DATA_BLOCK DB 6
TITLE =Codici trasferitore SALVARE PRIMA DEL DOWNLOAD
VERSION : 0.1


  STRUCT
   Codici : ARRAY  [0 .. 200 ] OF WORD ;
  END_STRUCT ;
BEGIN
   Codici[0] := W#16#FFFF;
   Codici[1] := W#16#FFFF;
   Codici[2] := W#16#DB;
   Codici[3] := W#16#FFFF;
   Codici[4] := W#16#4;
   Codici[5] := W#16#FFFF;
   Codici[6] := W#16#3;
   Codici[7] := W#16#DC;
   Codici[8] := W#16#9;
   Codici[9] := W#16#8;
   Codici[10] := W#16#D9;
   Codici[11] := W#16#0;
   Codici[12] := W#16#DA;
   Codici[13] := W#16#0;
   Codici[14] := W#16#0;
   Codici[15] := W#16#0;
   Codici[16] := W#16#0;
   Codici[17] := W#16#0;
   Codici[18] := W#16#0;
   Codici[19] := W#16#0;
   Codici[20] := W#16#0;
   Codici[21] := W#16#0;
   Codici[22] := W#16#0;
   Codici[23] := W#16#0;
   Codici[24] := W#16#0;
   Codici[25] := W#16#0;
   Codici[26] := W#16#0;
   Codici[27] := W#16#0;
   Codici[28] := W#16#0;
   Codici[29] := W#16#0;
   Codici[30] := W#16#0;
   Codici[31] := W#16#0;
   Codici[32] := W#16#0;
   Codici[33] := W#16#0;
   Codici[34] := W#16#0;
   Codici[35] := W#16#0;
   Codici[36] := W#16#0;
   Codici[37] := W#16#0;
   Codici[38] := W#16#0;
   Codici[39] := W#16#0;
   Codici[40] := W#16#0;
   Codici[41] := W#16#0;
   Codici[42] := W#16#0;
   Codici[43] := W#16#0;
   Codici[44] := W#16#0;
   Codici[45] := W#16#0;
   Codici[46] := W#16#0;
   Codici[47] := W#16#0;
   Codici[48] := W#16#0;
   Codici[49] := W#16#0;
   Codici[50] := W#16#0;
   Codici[51] := W#16#0;
   Codici[52] := W#16#0;
   Codici[53] := W#16#0;
   Codici[54] := W#16#0;
   Codici[55] := W#16#0;
   Codici[56] := W#16#0;
   Codici[57] := W#16#0;
   Codici[58] := W#16#0;
   Codici[59] := W#16#0;
   Codici[60] := W#16#0;
   Codici[61] := W#16#0;
   Codici[62] := W#16#0;
   Codici[63] := W#16#0;
   Codici[64] := W#16#0;
   Codici[65] := W#16#0;
   Codici[66] := W#16#0;
   Codici[67] := W#16#0;
   Codici[68] := W#16#0;
   Codici[69] := W#16#0;
   Codici[70] := W#16#0;
   Codici[71] := W#16#0;
   Codici[72] := W#16#0;
   Codici[73] := W#16#0;
   Codici[74] := W#16#0;
   Codici[75] := W#16#0;
   Codici[76] := W#16#0;
   Codici[77] := W#16#0;
   Codici[78] := W#16#0;
   Codici[79] := W#16#0;
   Codici[80] := W#16#0;
   Codici[81] := W#16#0;
   Codici[82] := W#16#0;
   Codici[83] := W#16#0;
   Codici[84] := W#16#0;
   Codici[85] := W#16#0;
   Codici[86] := W#16#0;
   Codici[87] := W#16#0;
   Codici[88] := W#16#0;
   Codici[89] := W#16#0;
   Codici[90] := W#16#0;
   Codici[91] := W#16#0;
   Codici[92] := W#16#0;
   Codici[93] := W#16#0;
   Codici[94] := W#16#0;
   Codici[95] := W#16#0;
   Codici[96] := W#16#0;
   Codici[97] := W#16#0;
   Codici[98] := W#16#0;
   Codici[99] := W#16#0;
   Codici[100] := W#16#0;
   Codici[101] := W#16#0;
   Codici[102] := W#16#0;
   Codici[103] := W#16#0;
   Codici[104] := W#16#0;
   Codici[105] := W#16#0;
   Codici[106] := W#16#0;
   Codici[107] := W#16#0;
   Codici[108] := W#16#0;
   Codici[109] := W#16#0;
   Codici[110] := W#16#0;
   Codici[111] := W#16#0;
   Codici[112] := W#16#0;
   Codici[113] := W#16#0;
   Codici[114] := W#16#0;
   Codici[115] := W#16#0;
   Codici[116] := W#16#0;
   Codici[117] := W#16#0;
   Codici[118] := W#16#0;
   Codici[119] := W#16#0;
   Codici[120] := W#16#0;
   Codici[121] := W#16#0;
   Codici[122] := W#16#0;
   Codici[123] := W#16#0;
   Codici[124] := W#16#0;
   Codici[125] := W#16#0;
   Codici[126] := W#16#0;
   Codici[127] := W#16#0;
   Codici[128] := W#16#0;
   Codici[129] := W#16#0;
   Codici[130] := W#16#0;
   Codici[131] := W#16#0;
   Codici[132] := W#16#0;
   Codici[133] := W#16#0;
   Codici[134] := W#16#0;
   Codici[135] := W#16#0;
   Codici[136] := W#16#0;
   Codici[137] := W#16#0;
   Codici[138] := W#16#0;
   Codici[139] := W#16#0;
   Codici[140] := W#16#0;
   Codici[141] := W#16#0;
   Codici[142] := W#16#0;
   Codici[143] := W#16#0;
   Codici[144] := W#16#0;
   Codici[145] := W#16#0;
   Codici[146] := W#16#0;
   Codici[147] := W#16#0;
   Codici[148] := W#16#0;
   Codici[149] := W#16#0;
   Codici[150] := W#16#0;
   Codici[151] := W#16#0;
   Codici[152] := W#16#0;
   Codici[153] := W#16#0;
   Codici[154] := W#16#0;
   Codici[155] := W#16#0;
   Codici[156] := W#16#0;
   Codici[157] := W#16#0;
   Codici[158] := W#16#0;
   Codici[159] := W#16#0;
   Codici[160] := W#16#0;
   Codici[161] := W#16#0;
   Codici[162] := W#16#0;
   Codici[163] := W#16#0;
   Codici[164] := W#16#0;
   Codici[165] := W#16#0;
   Codici[166] := W#16#0;
   Codici[167] := W#16#0;
   Codici[168] := W#16#0;
   Codici[169] := W#16#0;
   Codici[170] := W#16#0;
   Codici[171] := W#16#0;
   Codici[172] := W#16#0;
   Codici[173] := W#16#0;
   Codici[174] := W#16#0;
   Codici[175] := W#16#0;
   Codici[176] := W#16#0;
   Codici[177] := W#16#0;
   Codici[178] := W#16#0;
   Codici[179] := W#16#0;
   Codici[180] := W#16#0;
   Codici[181] := W#16#0;
   Codici[182] := W#16#0;
   Codici[183] := W#16#0;
   Codici[184] := W#16#0;
   Codici[185] := W#16#0;
   Codici[186] := W#16#0;
   Codici[187] := W#16#0;
   Codici[188] := W#16#0;
   Codici[189] := W#16#0;
   Codici[190] := W#16#0;
   Codici[191] := W#16#0;
   Codici[192] := W#16#0;
   Codici[193] := W#16#0;
   Codici[194] := W#16#0;
   Codici[195] := W#16#0;
   Codici[196] := W#16#0;
   Codici[197] := W#16#0;
   Codici[198] := W#16#0;
   Codici[199] := W#16#0;
   Codici[200] := W#16#0;
END_DATA_BLOCK

